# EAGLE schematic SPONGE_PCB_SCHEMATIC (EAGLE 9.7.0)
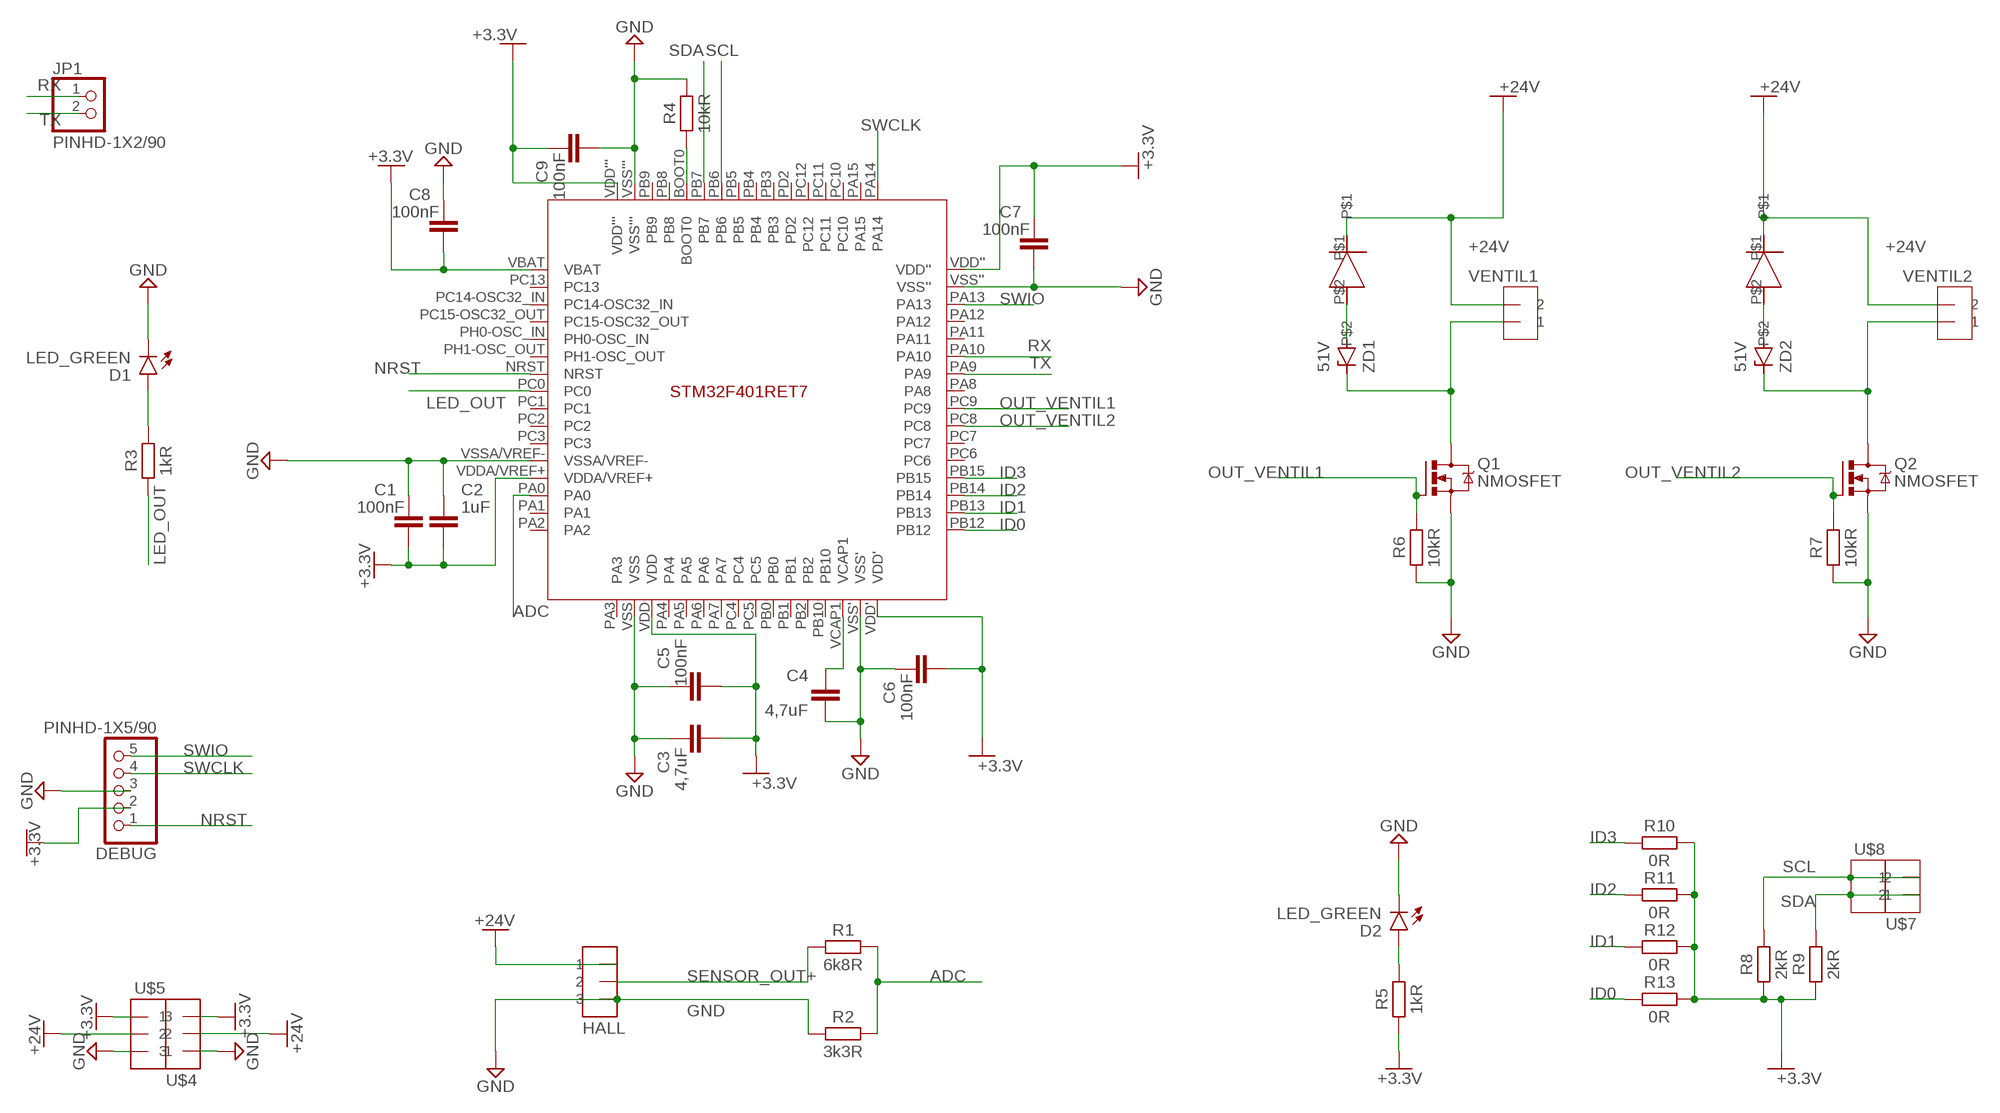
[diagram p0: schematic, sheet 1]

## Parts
C1  100nF  C_CHIP-0603(1608-METRIC)  [CAPC1608X85]
C2  1uF  C_CHIP-0603(1608-METRIC)  [CAPC1608X85]
C3  4,7uF  C_CHIP-0603(1608-METRIC)  [CAPC1608X85]
C4  4,7uF  C_CHIP-0603(1608-METRIC)  [CAPC1608X85]
C5  100nF  C_CHIP-0603(1608-METRIC)  [CAPC1608X85]
C6  100nF  C_CHIP-0603(1608-METRIC)  [CAPC1608X85]
C7  100nF  C_CHIP-0603(1608-METRIC)  [CAPC1608X85]
C8  100nF  C_CHIP-0603(1608-METRIC)  [CAPC1608X85]
C9  100nF  C_CHIP-0603(1608-METRIC)  [CAPC1608X85]
D1  LED_GREEN  CHIP-FLAT-G_1206  [LEDC3216X75N_FLAT-G]
D2  LED_GREEN  CHIP-FLAT-G_1206  [LEDC3216X75N_FLAT-G]
DEBUG  PINHD-1X5/90  [1X05/90]
HALL  FE3X1  [FE3X1]
JP1  PINHD-1X2/90  [1X02/90]
Q1  NMOSFET  NMOSFETSOT23-GSD  [SOT23]
Q2  NMOSFET  NMOSFETSOT23-GSD  [SOT23]
R1  6k8R  R_CHIP-1206(3216-METRIC)  [RESC3216X70]
R2  3k3R  R_CHIP-1206(3216-METRIC)  [RESC3216X70]
R3  1kR  R_CHIP-0603(1608-METRIC)  [RESC1608X60]
R4  10kR  R_CHIP-0603(1608-METRIC)  [RESC1608X60]
R5  1kR  R_CHIP-0603(1608-METRIC)  [RESC1608X60]
R6  10kR  R_CHIP-0603(1608-METRIC)  [RESC1608X60]
R7  10kR  R_CHIP-0603(1608-METRIC)  [RESC1608X60]
R8  2kR  R_CHIP-0603(1608-METRIC)  [RESC1608X60]
R9  2kR  R_CHIP-0603(1608-METRIC)  [RESC1608X60]
R10  0R  R_CHIP-0402(1005-METRIC)  [RESC1005X40]
R11  0R  R_CHIP-0402(1005-METRIC)  [RESC1005X40]
R12  0R  R_CHIP-0402(1005-METRIC)  [RESC1005X40]
R13  0R  R_CHIP-0402(1005-METRIC)  [RESC1005X40]
U$1  STM32F401RET7  [STM32F401_FOOTPRINT]
U$2  IN4005  [IN4005]
U$3  IN4005  [IN4005]
U$4  FE3X1  [FE3X1]
U$5  FE3X1  [FE3X1]
U$7  FE2X1  [FE2X1]
U$8  FE2X1  [FE2X1]
VENTIL1  FE2X1  [FE2X1]
VENTIL2  FE2X1  [FE2X1]
ZD1  51V  ZENER_1N4757  [ZENER_1N4757]
ZD2  51V  ZENER_1N4757  [ZENER_1N4757]

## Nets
+3.3V: C1.2 C2.2 C3.2 C5.2 C6.2 C7.1 C8.2 C9.1 DEBUG.2 R5.1 R8.1 R9.1 R10.2 R11.2 R12.2 R13.2 U$1.VBAT U$1.VDD U$1.VDD' U$1.VDD'' U$1.VDD''' U$1.VDDA/VREF+ U$4.P$1 U$5.P$3
+24V: HALL.P$1 U$2.P$1 U$3.P$1 U$4.P$2 U$5.P$2 VENTIL1.P$1 VENTIL2.P$1
ADC: R1.2 R2.2 U$1.PA0
GND: C1.1 C2.1 C3.1 C4.1 C5.1 C6.1 C7.2 C8.1 C9.2 D1.C D2.C DEBUG.3 HALL.P$3 Q1.2(S) Q2.2(S) R2.1 R4.2 R6.1 R7.1 U$1.VSS U$1.VSS' U$1.VSS'' U$1.VSS''' U$1.VSSA/VREF- U$4.P$3 U$5.P$1
ID0: R13.1 U$1.PB12
ID1: R12.1 U$1.PB13
ID2: R11.1 U$1.PB14
ID3: R10.1 U$1.PB15
LED_OUT: R3.1 U$1.PC0
N$1: C4.2 U$1.VCAP1
N$2: R4.1 U$1.BOOT0
N$3: D1.A R3.2
N$5: Q1.3(D) VENTIL1.P$2 ZD1.P$2(C)
N$6: Q2.3(D) VENTIL2.P$2 ZD2.P$2(C)
N$7: U$3.P$2 ZD2.P$1(A)
N$8: U$2.P$2 ZD1.P$1(A)
N$9: D2.A R5.2
NRST: DEBUG.1 U$1.NRST
OUT_VENTIL1: Q1.1(G) R6.2 U$1.PC9
OUT_VENTIL2: Q2.1(G) R7.2 U$1.PC8
RX: JP1.1 U$1.PA10
SCL: R8.2 U$1.PB6 U$7.P$2 U$8.P$1
SDA: R9.2 U$1.PB7 U$7.P$1 U$8.P$2
SENSOR_OUT+: HALL.P$2 R1.1
SWCLK: DEBUG.4 U$1.PA14
SWIO: DEBUG.5 U$1.PA13
TX: JP1.2 U$1.PA9
Unconnected: U$1.PA1 U$1.PA2 U$1.PA3 U$1.PA4 U$1.PA5 U$1.PA6 U$1.PA7 U$1.PA8 U$1.PA11 U$1.PA12 U$1.PA15 U$1.PB0 U$1.PB1 U$1.PB2 U$1.PB3 U$1.PB4 U$1.PB5 U$1.PB8 U$1.PB9 U$1.PB10 U$1.PC1 U$1.PC2 U$1.PC3 U$1.PC4 U$1.PC5 U$1.PC6 U$1.PC7 U$1.PC10 U$1.PC11 U$1.PC12 U$1.PC13 U$1.PC14-OSC32_IN U$1.PC15-OSC32_OUT U$1.PD2 U$1.PH0-OSC_IN U$1.PH1-OSC_OUT

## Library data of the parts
C1-C9 = Capacitor:C: Capacitor - Generic; CATEGORY: Capacitor
D1 D2 = LED:CHIP-FLAT-G; CATEGORY: LED; COLOR: GREEN; DESCRIPTION: CHIP LED FLAT; SUB-CATEGORY: CHIP; TYPE: FLAT_TOP
DEBUG = Connector:PINHD-1X5: PIN HEADER; CATEGORY: CONNECTOR; SUB-CATEGORY: PIN-HEADER
HALL U$4 U$5 = Haley_Components:FE3X1
JP1 = Connector:PINHD-1X2: PIN HEADER; CATEGORY: CONNECTOR; SUB-CATEGORY: PIN-HEADER
Q1 Q2 = Transistor:NMOSFET: N-Channel MOSFET - Generic; CATEGORY: Transistor; SUB-CATEGORY: MOSFET; TYPE: N-Channel
R1-R13 = Resistor:R: Resistor Fixed - Generic; CATEGORY: Resistor; SUB-CATEGORY: Fixed
U$1 = Haley_Components:STM32F401RET7
U$2 U$3 = Haley_Components:IN4005
U$7 U$8 VENTIL1 VENTIL2 = Haley_Components:FE2X1
ZD1 ZD2 = Haley_Components:ZENER_1N4757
